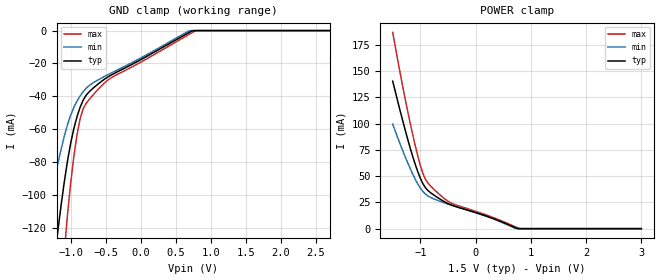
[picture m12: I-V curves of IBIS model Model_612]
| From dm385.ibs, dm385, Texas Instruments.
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| Model based on original model for BCSHTLTCSCDDVPBFZ_SSDHV
|   Sub model DIFF_VREF_FULLTERM_10MA_5PER_1P5
[model]   Model_612
|[Description]  [1.5V-INPUT-FULLTERM:10MA-X, IND, 5%]
|   FULLTERM, 0.80 * RExt = 1.250 * Iout (I[2:0] = "101"), 10mA
|   nominal with Rext = 50R,Industrial temperature range (-40C to
|   125C, 25C nominal),5% power supply tolerance
|[Input Load]   FULLTERM:10MA
|[Output Drive]
|Voltage   1.5V
|Mode   INPUT
Model_type   Input
Polarity   Non-Inverting
Vinl =  0.65
Vinh =  0.85
C_comp   1.865048p   1.679967p   1.989968p
[Model Spec]
Vinl   0.65   0.6125   0.6875
Vinh   0.85   0.8125   0.8875
[Temperature Range]   25   125   -40
[Voltage Range]   1.5   1.425   1.575
[POWER_clamp]
-1.5V     140.4mA    99.41mA    186.8mA
-1.227V   84.83mA    62.51mA    111.3mA
-1.091V   60.98mA    46.94mA    78.75mA
-1V       48mA       38.63mA    60.16mA
-954.5mV  42.92mA    35.44mA    52.69mA
-863.6mV  36.35mA    31.19mA    43.46mA
-545.5mV  25.1mA     24.25mA    27.81mA
-409.1mV  21.86mA    21.97mA    23.58mA
181.8mV   12.14mA    12.16mA    13.23mA
727.3mV   768.4uA    61.12uA    1.508mA
818.2mV   0A         0A         0A
3V        0A         0A         0A
[GND_clamp]
-1.5V     -241.5mA   -151.1mA   -386.7mA
-1.364V   -188.6mA   -119.8mA   -299mA
-1.182V   -122mA     -81.04mA   -186.4mA
-1.091V   -92.47mA   -64.48mA   -135.3mA
-1.045V   -79.75mA   -57.51mA   -112.9mA
-1V       -68.87mA   -51.64mA   -93.45mA
-909.1mV  -52.51mA   -42.95mA   -63.65mA
-863.6mV  -46.63mA   -39.74mA   -53.56mA
-681.8mV  -35.14mA   -31.85mA   -39.3mA
-409.1mV  -26.76mA   -25.55mA   -28.4mA
772.7mV   0A         0A         -294.4uA
3V        0A         0A         0A
